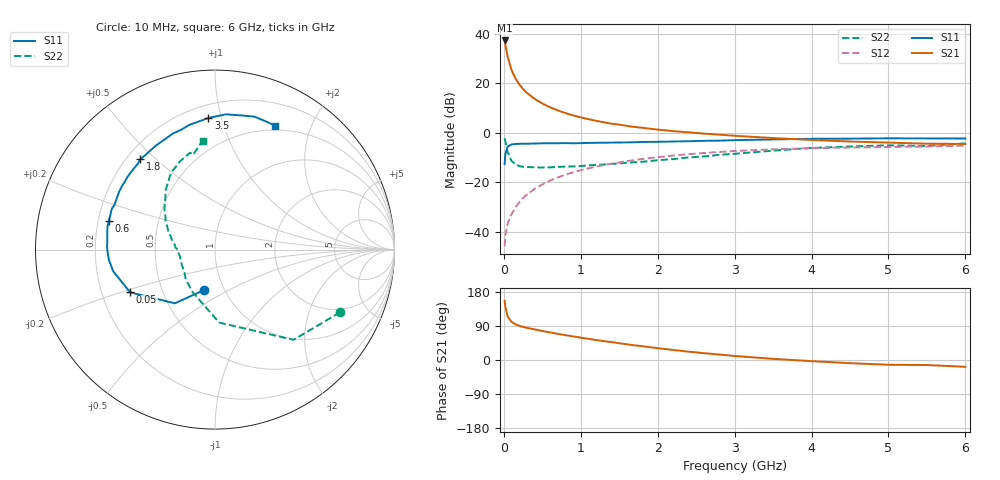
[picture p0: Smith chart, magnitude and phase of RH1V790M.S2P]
! SIEMENS Small Signal Semiconductors
! BFR106
! Si NPN RF Bipolar Junction Transistor in SOT23
! VCE = 1.75 V  IC = 90 mA
! Common Emitter S-Parameters:  August  1996
# GHz  S  MA  R  50
!  f  S11  S21  S12  S22
! GHz  MAG  ANG  MAG  ANG  MAG  ANG  MAG  ANG
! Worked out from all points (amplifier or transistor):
!   36 points, 10 MHz to 6 GHz, reference 50 ohm
!   highest |S21| = 37.3 dB at 10 MHz (marker M1)
!   |S21| within 3 dB of that: start of sweep to 27.94 MHz
!   unconditionally stable (mu >= 1): 132.3 MHz to end of sweep
!   at 250 MHz: K = 1.10, MAG = 20.1 dB, |S12| = -26.4 dB
!   at 1.4 GHz: K = 1.09, MAG = 6.2 dB, |S12| = -12.5 dB
!   at 6 GHz: K = 1.02, MAG = -0.6 dB, |S12| = -5.2 dB
!   S11 on the Smith chart (normalised r, x): 10 MHz: 0.81, -0.38; 50 MHz: 0.32, -0.21; 600 MHz: 0.24, +0.12; 1.8 GHz: 0.25, +0.45; 3.5 GHz: 0.29, +0.91; 6 GHz: 0.45, +1.51
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0.01  0.2328 -104.9  73.58 156.7  0.0051 71.8  0.7798 -26.6
0.02  0.3739 -126.8  60.56 139.6  0.0085 64.6  0.6661 -49.0
0.05  0.5293 -153.3  34.28 114.7  0.0148 59.6  0.4074 -86.7
0.1  0.58 -168.0  18.67 100.7  0.0227 65.1  0.2687 -117.2
0.15  0.5937 -174.4  12.64 94.3  0.031 68.5  0.2339 -134.0
0.2  0.5982 -178.3  9.59 90.4  0.0391 70.8  0.212 -143.3
0.25  0.6018 178.4  7.669 87.2  0.0478 71.8  0.2052 -151.5
0.3  0.601 176.5  6.416 84.9  0.0564 73.1  0.2033 -155.8
0.4  0.6066 171.9  4.855 80.7  0.0736 73.2  0.2002 -163.3
0.5  0.6123 168.1  3.911 76.6  0.0905 72.5  0.1984 -168.3
0.6  0.6127 164.9  3.284 72.8  0.108 71.5  0.2001 -171.1
0.7  0.6144 161.5  2.842 68.9  0.125 70.1  0.2043 -174.2
0.8  0.6181 158.6  2.502 65.6  0.1417 68.5  0.2074 -177.1
1.1  0.6242 148.8  1.886 55.9  0.1912 63.9  0.2201 176.9
1.4  0.634 140.5  1.53 47.2  0.2374 58.4  0.2344 170.7
1.8  0.6537 129.5  1.263 36.4  0.2945 51.3  0.2593 162.7
2.2  0.6665 119.6  1.081 26.5  0.3465 44.1  0.2939 154.5
3  0.7091 101.7  0.87 10.6  0.4277 30.3  0.3764 138.0
3.5  0.7343 92.9  0.782 3.0  0.4642 22.5  0.4354 128.8
4.5  0.7615 79.1  0.666 -8.4  0.5037 8.3  0.5289 111.6
5.5  0.7684 68.0  0.602 -13.3  0.5262 -0.1  0.5414 103.1
6  0.7674 64.0  0.596 -18.0  0.5512 -6.7  0.6107 96.5
